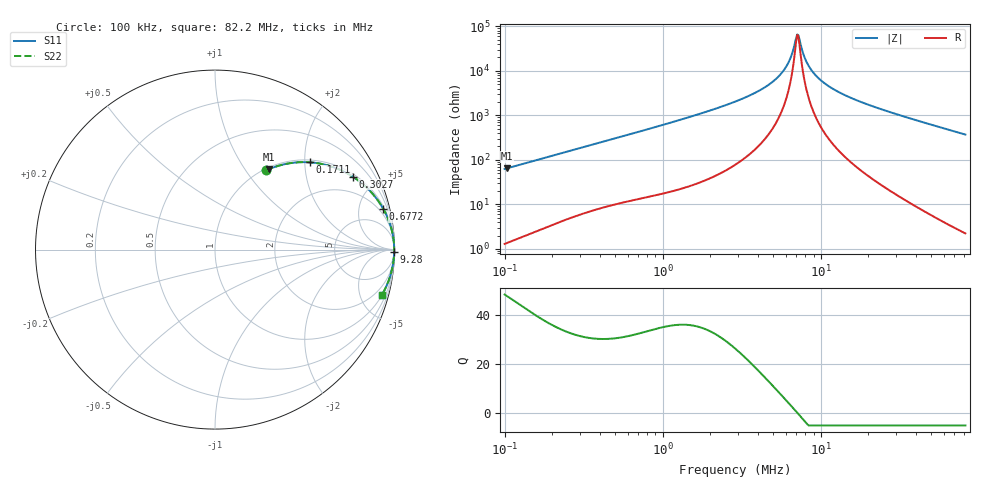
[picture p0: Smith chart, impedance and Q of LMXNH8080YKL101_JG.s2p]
! LMXNH8080YKL101_JG  S-PARAMETER MODEL  ( General Type )
! Model Generated by TAIYO YUDEN Corporation (http://www.ty-top.com)
! Version 1.0
! TAIYO YUDEN Control No. 191025NI43SB-FBB
! Copyright(c) 2019 TAIYO YUDEN CO.,LTD. All Rights Reserved.
! Product Description (link to TY-COMPAS)
! https://ds.yuden.co.jp/TYCOMPAS/or/detail?pn=LMXNH8080YKL101MJG&u=M
! Products Name : Inductors
! Characteristics :
!  Inductance : 100 uH , SRF(min) : 6.0 MHz , DC Resistance(max) : 0.364 Ohm
!  Rated Current : Saturation :1100 mA , Temp Rise : 1000 mA
!  Case Size : 8.0 x 8.0 / 0.315 x 0.315 [mm/inch] , Thickness : 4 / 0.157 [mm/inch]
!  (Conditions: Temperature = 25 degC , DC Bias Current/Voltage = 0A / 0V)
! External Node Assignments :
!  1  o---GGG---o  2
! GND o---------o GND
! Frequency Range : 0.1MHz  -  82.198079MHz  [ 402 STEP ]
# MHz S RI R 50
! Freq[MHz].  S11 Real  S11 Imag  S21 Real  S21 Imag  S12 Real  S12 Imag  S22 Real  S22 Imag
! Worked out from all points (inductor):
!   401 points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, 100 kHz to 82.2 MHz, reference 50 ohm
!   read as one part in series: L = 99.1 uH near 103.4 kHz
!   highest Q = 47.5 at 103.4 kHz (marker M1), where L = 99.4 uH
!   self-resonance near 7.095 MHz
!   S11 on the Smith chart (normalised r, x): 100 kHz: 1.03, +1.25; 171.1 kHz: 1.06, +2.12; 302.7 kHz: 1.12, +3.72; 677.2 kHz: 1.26, +8.20; 9.28 MHz: open; 82.2 MHz: 1.04, -7.40
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0.1  0.2848 0.441  0.7152 -0.441  0.7152 -0.441  0.2848 0.441
0.103413  0.2983 0.4471  0.7017 -0.4471  0.7017 -0.4471  0.2983 0.4471
0.171076  0.5294 0.4862  0.4706 -0.4862  0.4706 -0.4862  0.5294 0.4862
0.302658  0.7683 0.4062  0.2317 -0.4062  0.2317 -0.4062  0.7683 0.4062
0.307779  0.7739 0.4025  0.2261 -0.4025  0.2261 -0.4025  0.7739 0.4025
0.677229  0.9376 0.2267  0.0624 -0.2267  0.0624 -0.2267  0.9376 0.2267
0.947281  0.9661 0.167  0.0339 -0.167  0.0339 -0.167  0.9661 0.167
2.867021  0.9957 0.0491  0.00429 -0.0491  0.00429 -0.0491  0.9957 0.0491
4.217309  0.9977 0.026  0.00231 -0.026  0.00231 -0.026  0.9977 0.026
5.424287  0.9983 0.0131  0.00172 -0.0131  0.00172 -0.0131  0.9983 0.0131
6.203545  0.9984 0.00665  0.00157 -0.00665  0.00157 -0.00665  0.9984 0.00665
6.523811  0.9985 0.00426  0.00153 -0.00426  0.00153 -0.00426  0.9985 0.00426
6.976699  0.9985 0.00109  0.0015 -0.00109  0.0015 -0.00109  0.9985 0.00109
7.094751  0.9985 0.000295  0.0015 -0.000295  0.0015 -0.000295  0.9985 0.000295
7.336881  0.9985 -0.00129  0.0015 0.00129  0.0015 0.00129  0.9985 -0.00129
8.113989  0.9985 -0.00605  0.00152 0.00605  0.00152 0.00605  0.9985 -0.00605
8.824095  0.9984 -0.0101  0.00158 0.0101  0.00158 0.0101  0.9984 -0.0101
9.279651  0.9984 -0.0125  0.00163 0.0125  0.00163 0.0125  0.9984 -0.0125
10.97497  0.9981 -0.0209  0.0019 0.0209  0.0019 0.0209  0.9981 -0.0209
13.65011  0.9975 -0.0327  0.00252 0.0327  0.00252 0.0327  0.9975 -0.0327
27.15873  0.9916 -0.083  0.00839 0.083  0.00839 0.083  0.9916 -0.083
82.19808  0.9306 -0.2512  0.0694 0.2512  0.0694 0.2512  0.9306 -0.2512
